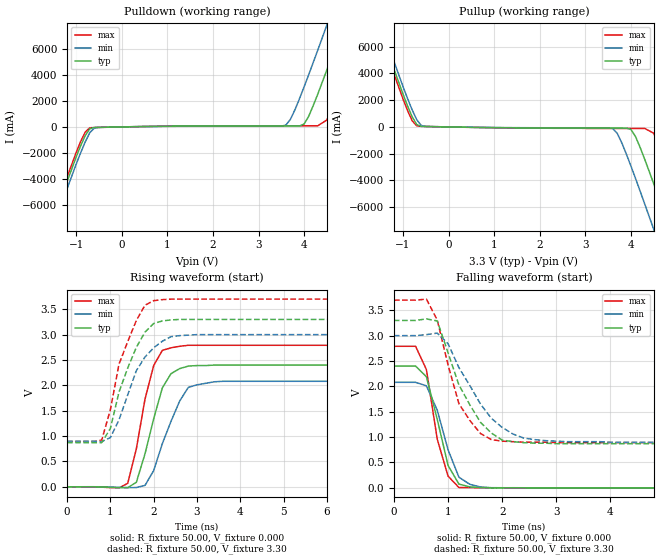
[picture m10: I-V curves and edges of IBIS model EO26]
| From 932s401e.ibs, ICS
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|   Model EO26
[Model]   EO26
Model_type   Output
Polarity   Non-Inverting
C_comp   2.50pF   2.00pF   3.00pF
[Temperature Range]   27.00   70.00   0.000
[Voltage Range]   3.30V   3.00V   3.70V
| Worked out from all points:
|   slope of the pulldown table from 0 to 0.495 V, typ, clamps not added: 15.9 ohm
|   slope of the pullup table from 0 to 0.495 V, typ, clamps not added: 17.1 ohm
|   rising waveform, R_fixture 50.00, V_fixture 0.000: 20-80 % time 451ps typ, 551ps min, 408ps max; typ from 0 V to 2.4 V
|   rising waveform, R_fixture 50.00, V_fixture 3.30: 20-80 % time 585ps typ, 622ps min, 555ps max; typ from 0.87 V to 3.3 V
|   falling waveform, R_fixture 50.00, V_fixture 0.000: 20-80 % time 327ps typ, 380ps min, 296ps max; typ from 2.4 V to 0 V
|   falling waveform, R_fixture 50.00, V_fixture 3.30: 20-80 % time 611ps typ, 745ps min, 487ps max; typ from 3.3 V to 0.87 V
[Pulldown]
| voltage   I(typ)   I(min)   I(max)
-3.3V     -24.68A    -25.4A     -24.36A
-1.7V     -8.95A     -9.49A     -8.61A
-1.5V     -7.01A     -7.56A     -6.67A
-900mV    -1.43A     -1.96A     -1.1A
-700mV    -140mA     -430mA     -67.64mA
3.6V      70.25mA    140mA      86.6mA
4V        220mA      3.07A      86.87mA
4.3V      2.51A      5.88A      87.78mA
4.5V      4.37A      7.81A      530mA
4.9V      8.22A      11.69A     4.03A
5.3V      12.13A     15.62A     7.88A
6.6V      24.98A     28.48A     20.69A
[Pullup]
| voltage   I(typ)   I(min)   I(max)
-3.3V     24.83A     25.37A     24.5A
-1.7V     9.09A      9.66A      8.74A
-1.5V     7.16A      7.73A      6.8A
-900mV    1.56A      2.11A      1.21A
-700mV    180mA      540mA      80.2mA
3.6V      -85.86mA   -120mA     -110mA
4V        -190mA     -2.93A     -110mA
4.3V      -2.4A      -5.74A     -110mA
4.5V      -4.25A     -7.66A     -470mA
4.9V      -8.1A      -11.56A    -3.93A
5.3V      -12.02A    -15.49A    -7.78A
6.6V      -24.89A    -28.38A    -20.62A
[Ramp]
| variable   typ   min   max
dV/dt_r   1.44/0.43n   1.25/0.55n   1.67/0.38n
dV/dt_f   1.46/0.54n   1.26/0.68n   1.68/0.45n
R_load = 50.00
[Rising Waveform]
R_fixture = 50.00
V_fixture = 0.000
V_fixture_min = 0.000
V_fixture_max = 0.000
| time   V(typ)   V(min)   V(max)
0s        0V         0V         0V
1.4ns     -18.1mV    -16.25mV   67.28mV
1.6ns     88.87mV    -15.26mV   750mV
1.8ns     650mV      27.23mV    1.73V
2ns       1.34V      320mV      2.39V
2.2ns     1.95V      850mV      2.69V
2.6ns     2.33V      1.69V      2.77V
2.8ns     2.38V      1.96V      2.79V
3ns       2.39V      2.01V      2.79V
10ns      2.4V       2.08V      2.79V
[Rising Waveform]
R_fixture = 50.00
V_fixture = 3.30
V_fixture_min = 3.00
V_fixture_max = 3.70
| time   V(typ)   V(min)   V(max)
0s        870mV      900mV      890mV
800ps     870mV      890mV      920mV
1ns       1.15V      970mV      1.52V
1.2ns     1.87V      1.32V      2.42V
1.6ns     2.75V      2.29V      3.28V
1.8ns     3.05V      2.56V      3.58V
2ns       3.22V      2.74V      3.67V
2.4ns     3.29V      2.96V      3.7V
3ns       3.3V       3V         3.7V
10ns      3.3V       3V         3.7V
[Falling Waveform]
R_fixture = 50.00
V_fixture = 0.000
V_fixture_min = 0.000
V_fixture_max = 0.000
| time   V(typ)   V(min)   V(max)
0s        2.4V       2.08V      2.79V
400ps     2.4V       2.08V      2.79V
600ps     2.19V      2.01V      2.33V
800ps     1.35V      1.53V      960mV
1ns       440mV      750mV      230mV
1.2ns     73.77mV    210mV      6.53mV
1.4ns     18.65mV    69.7mV     3.11mV
1.6ns     4.86mV     16.42mV    1.67mV
1.8ns     -830uV     2.21mV     720uV
10ns      9.75uV     11.14uV    0V
[Falling Waveform]
R_fixture = 50.00
V_fixture = 3.30
V_fixture_min = 3.00
V_fixture_max = 3.70
| time   V(typ)   V(min)   V(max)
0s        3.3V       3V         3.7V
600ps     3.33V      3.02V      3.72V
800ps     3.29V      3.05V      3.31V
1ns       2.66V      2.84V      2.42V
1.2ns     2.03V      2.37V      1.66V
1.6ns     1.29V      1.65V      1.07V
1.8ns     1.08V      1.37V      950mV
2.2ns     910mV      1.06V      910mV
2.8ns     880mV      930mV      900mV
10ns      870mV      900mV      890mV
